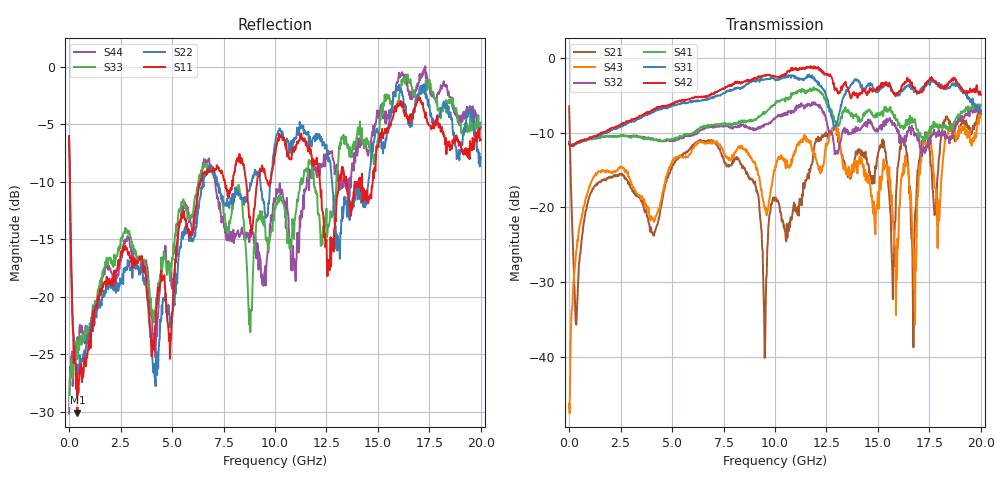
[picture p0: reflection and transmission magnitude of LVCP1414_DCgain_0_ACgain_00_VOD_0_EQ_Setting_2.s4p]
!Agilent Technologies,N5230A,MY46400459,A.07.50.48
!Agilent N5230A: A.07.50.48
!Date: Tuesday, April 17, 2012 18:34:04
!Correction: S11(Full 4 Port(1,2,3,4))
!S12(Full 4 Port(1,2,3,4))
!S13(Full 4 Port(1,2,3,4))
!S14(Full 4 Port(1,2,3,4))
!S21(Full 4 Port(1,2,3,4))
!S22(Full 4 Port(1,2,3,4))
!S23(Full 4 Port(1,2,3,4))
!S24(Full 4 Port(1,2,3,4))
!S31(Full 4 Port(1,2,3,4))
!S32(Full 4 Port(1,2,3,4))
!S33(Full 4 Port(1,2,3,4))
!S34(Full 4 Port(1,2,3,4))
!S41(Full 4 Port(1,2,3,4))
!S42(Full 4 Port(1,2,3,4))
!S43(Full 4 Port(1,2,3,4))
!S44(Full 4 Port(1,2,3,4))
!S4P File: Measurements: <S11,S12,S13,S14>,
!<S21,S22,S23,S24>,
!<S31,S32,S33,S34>,
!<S41,S42,S43,S44>:
# Hz S  dB  R 50
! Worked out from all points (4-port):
!   801 points, 300 kHz to 20 GHz, reference 50 ohm
!   strongest paths, dB at 300 kHz, 5 GHz, 10 GHz, 15 GHz, 20 GHz:
!     S42: -11.4, -6.1, -2.5, -3.9, -4.9
!     S31: -11.2, -6.4, -2.9, -4.5, -7.4
!     S41: -11.3, -10.7, -6.2, -7.3, -6.3
!     S32: -11.4, -11.1, -8.1, -9.9, -7.0
!     S43: -46.3, -13.9, -15.0, -17.9, -7.3
!     S21: -6.4, -14.5, -19.1, -12.9, -7.3
!   lowest |S11| = -30.1 dB at 400.3 MHz (marker M1), VSWR 1.06, Z = 52.9 + j1.36 ohm
!   |S11| at or under -10 dB: 37.64 MHz to 6.381 GHz (6.344 GHz wide, 198 % of centre); 8.602 GHz to 9.135 GHz (533.1 MHz wide, 6.01 % of centre); 12.18 GHz to 13.1 GHz (917.6 MHz wide, 7.26 % of centre)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
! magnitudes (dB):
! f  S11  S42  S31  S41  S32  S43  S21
! 300 kHz  -6.0  -11.4  -11.2  -11.3  -11.4  -46.3  -6.4
! 400.3 MHz  -30.1  -11.2  -11.2  -11.3  -11.3  -24.3  -32.2
! 9.9 GHz  -8.6  -2.3  -2.6  -6.3  -8.3  -15.9  -18.7
! 12.75 GHz  -15.0  -2.5  -8.0  -6.9  -10.1  -9.9  -10.1
! 14 GHz  -10.1  -5.3  -2.9  -7.8  -9.3  -15.4  -12.9
! 16.8 GHz  -3.5  -3.9  -4.2  -8.2  -10.0  -35.7  -21.1
! 20 GHz  -6.3  -4.9  -7.4  -6.3  -7.0  -7.3  -7.3
